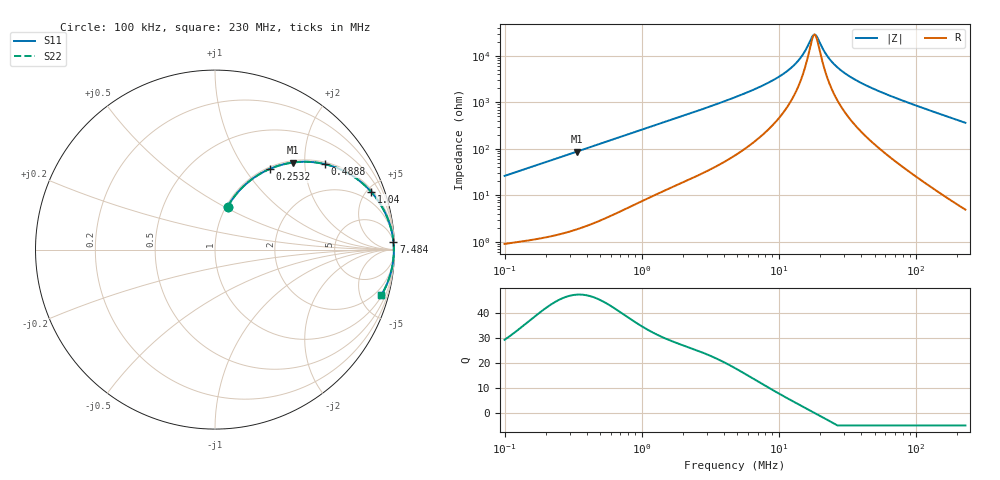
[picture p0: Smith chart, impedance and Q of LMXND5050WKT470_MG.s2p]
! LMXND5050WKT470_MG  S-PARAMETER MODEL  ( General Type )
! Model Generated by TAIYO YUDEN Corporation (https://www.yuden.co.jp/en/)
! Version 1.0
! TAIYO YUDEN Control No. 191023NI43SB-FBB
! Copyright(c) 2019 TAIYO YUDEN CO.,LTD. All Rights Reserved.
! Product Description (link to TY-COMPAS)
! https://ds.yuden.co.jp/TYCOMPAS/or/detail?pn=LMXND5050WKT470MMG&u=M
! Products Name : Inductors
! Characteristics :
!  Inductance : 47 uH , SRF(min) : 12 MHz , DC Resistance(max) : 0.522 Ohm
!  Rated Current : Saturation :630 mA , Temp Rise : 560 mA (40 degC)
!  Case Size : 4.9 x 4.9 / 0.193 x 0.193 [mm/inch] , Thickness : 2 / 0.079 [mm/inch]
!  (Conditions: Temperature = 25 degC , DC Bias Current/Voltage = 0A / 0V)
! External Node Assignments :
!  1  o---GGG---o  2
! GND o---------o GND
! Frequency Range : 0.1MHz  -  229.966873MHz  [ 402 STEP ]
# MHz S RI R 50
! Freq[MHz].  S11 Real  S11 Imag  S21 Real  S21 Imag  S12 Real  S12 Imag  S22 Real  S22 Imag
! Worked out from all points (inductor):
!   401 points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, 100 kHz to 230 MHz, reference 50 ohm
!   read as one part in series: L = 41.4 uH near 103.9 kHz
!   highest Q = 47.1 at 338.4 kHz (marker M1), where L = 41.1 uH
!   self-resonance near 18.23 MHz
!   S11 on the Smith chart (normalised r, x): 100 kHz: 1.02, +0.52; 253.2 kHz: 1.03, +1.31; 488.8 kHz: 1.06, +2.52; 1.04 MHz: 1.16, +5.33; 7.484 MHz: 5, +45; 230 MHz: 1.10, -7.26
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0.1  0.0709 0.2401  0.9291 -0.2401  0.9291 -0.2401  0.0709 0.2401
0.16222  0.157 0.3509  0.843 -0.3509  0.843 -0.3509  0.157 0.3509
0.253163  0.3042 0.4492  0.6958 -0.4492  0.6958 -0.4492  0.3042 0.4492
0.338425  0.4347 0.4852  0.5653 -0.4852  0.5653 -0.4852  0.4347 0.4852
0.365661  0.4721 0.4887  0.5279 -0.4887  0.5279 -0.4887  0.4721 0.4887
0.488811  0.6114 0.4765  0.3886 -0.4765  0.3886 -0.4765  0.6114 0.4765
0.719821  0.7686 0.4093  0.2314 -0.4093  0.2314 -0.4093  0.7686 0.4093
1.03969  0.8695 0.3224  0.1305 -0.3224  0.1305 -0.3224  0.8695 0.3224
1.337081  0.9141 0.2645  0.0859 -0.2645  0.0859 -0.2645  0.9141 0.2645
4.889189  0.99 0.0748  0.00995 -0.0748  0.00995 -0.0748  0.99 0.0748
7.483907  0.9943 0.0441  0.00574 -0.0441  0.00574 -0.0441  0.9943 0.0441
10.19988  0.9957 0.0268  0.00432 -0.0268  0.00432 -0.0268  0.9957 0.0268
12.86604  0.9962 0.0156  0.00376 -0.0156  0.00376 -0.0156  0.9962 0.0156
15.02029  0.9964 0.00854  0.00355 -0.00854  0.00355 -0.00854  0.9964 0.00854
17.53523  0.9965 0.00173  0.00345 -0.00173  0.00345 -0.00173  0.9965 0.00173
18.2272  0.9966 4.36e-05  0.00344 -4.36e-05  0.00344 -4.36e-05  0.9966 4.36e-05
18.94647  0.9966 -0.00165  0.00344 0.00165  0.00344 0.00165  0.9966 -0.00165
22.99163  0.9965 -0.0102  0.00352 0.0102  0.00352 0.0102  0.9965 -0.0102
29.00146  0.9962 -0.021  0.00384 0.021  0.00384 0.021  0.9962 -0.021
40.29866  0.9951 -0.0383  0.00487 0.0383  0.00487 0.0383  0.9951 -0.0383
64.11956  0.9916 -0.0702  0.00837 0.0702  0.00837 0.0702  0.9916 -0.0702
229.9669  0.9265 -0.2542  0.0735 0.2542  0.0735 0.2542  0.9265 -0.2542
